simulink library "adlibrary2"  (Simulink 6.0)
settings: Solver=ode45  StartTime=0.0  StopTime=10.0  RelTol=1e-3
undefined symbols (not defined in the file or in its folder): adlibrary2, ADM, Bit, DDR, Generation, II, Location, Lower, SDRAM, SRAM, Width, XP, XPL, XRC, ZBT
libraries: xbsIndex_r3 x581, adlibrary2 x2
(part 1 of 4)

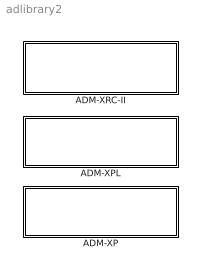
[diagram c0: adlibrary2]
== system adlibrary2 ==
  ADM-XP : Subsystem
  ADM-XPL : Subsystem
  ADM-XRC-II : Subsystem

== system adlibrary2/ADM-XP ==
  DDR SDRAM 1 : Subsystem  mask{memsize=1}
      mask prompts: memsize "Simulation RAM Size (Mb)"
      mask init:
      | as=get_param(gcb,'MaskIconUnits');
      | if (as(1)=='p')
      | 	im=imread('adbutton.jpg');s=get_param(gcb,'MaskDisplay');
      |     add_ad_icon(67,60);
      | else	
      | 	rm_ad_icon
      | end
  DDR SDRAM 2 : Subsystem  AncestorBlock=adlibrary2/ADM-XP/DDR SDRAM 1  mask{memsize=1}
      mask prompts: memsize "Simulation RAM Size (Mb)"
      mask init:
      | as=get_param(gcb,'MaskIconUnits');
      | if (as(1)=='p')
      | 	im=imread('adbutton.jpg');s=get_param(gcb,'MaskDisplay');
      |     add_ad_icon(67,60);
      | else	
      | 	rm_ad_icon
      | end
  DDRII SRAM 0 : Subsystem
  DDRII SRAM 1 : Subsystem
  DDRII SRAM 2 : Subsystem
  DDRII SRAM 3 : Subsystem
  XPL 32 Bit Interface : Subsystem  mask{program='load myprogram.txt', clock_ratio=1.5}
      mask prompts: program "Local Bus Script Program"; clock_ratio "Clock Ratio"
      mask init:
      | as=get_param(gcb,'MaskIconUnits');
      | if (as(1)=='p')
      | 	im=imread('adbutton.jpg');s=get_param(gcb,'MaskDisplay');
      |     add_ad_icon(74,56);
      | else	
      | 	rm_ad_icon
      | end
  XPL 64 Bit Interface : Subsystem  mask{program='load myprogram.txt', clock_ratio=1.5}
      mask prompts: program "Local Bus Script Program"; clock_ratio "Clock Ratio"
      mask init:
      | as=get_param(gcb,'MaskIconUnits');
      | if (as(1)=='p')
      | 	im=imread('adbutton.jpg');s=get_param(gcb,'MaskDisplay');
      |     add_ad_icon(74,56);
      | else	
      | 	rm_ad_icon
      | end

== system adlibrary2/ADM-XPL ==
  "DDR SDRAM " : Subsystem  mask{memsize=1}
      mask prompts: memsize "Simulation RAM Size (Mb)"
      mask init:
      | as=get_param(gcb,'MaskIconUnits');
      | if (as(1)=='p')
      | 	im=imread('adbutton.jpg');s=get_param(gcb,'MaskDisplay');
      |     add_ad_icon(67,60);
      | else	
      | 	rm_ad_icon
      | end
  XPL 32 Bit Interface : Subsystem  mask{program='load myprogram.txt', clock_ratio=1.5}
      mask prompts: program "Local Bus Script Program"; clock_ratio "Clock Ratio"
      mask init:
      | as=get_param(gcb,'MaskIconUnits');
      | if (as(1)=='p')
      | 	im=imread('adbutton.jpg');s=get_param(gcb,'MaskDisplay');
      |     add_ad_icon(74,56);
      | else	
      | 	rm_ad_icon
      | end
  XPL 64 Bit Interface : Subsystem  mask{program='load myprogram.txt', clock_ratio=1.5}
      mask prompts: program "Local Bus Script Program"; clock_ratio "Clock Ratio"
      mask init:
      | as=get_param(gcb,'MaskIconUnits');
      | if (as(1)=='p')
      | 	im=imread('adbutton.jpg');s=get_param(gcb,'MaskDisplay');
      |     add_ad_icon(74,56);
      | else	
      | 	rm_ad_icon
      | end
  ZBT SRAM 64 : Subsystem

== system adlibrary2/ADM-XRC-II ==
  PLX 32 Bit Interface : Subsystem  mask{program='load myprogram.txt', clock_ratio=1.5}
      mask prompts: program "Local Bus Script Program"; clock_ratio "Clock Ratio"
      mask init:
      | as=get_param(gcb,'MaskIconUnits');
      | if (as(1)=='p')
      | 	im=imread('adbutton.jpg');s=get_param(gcb,'MaskDisplay');
      |     add_ad_icon(74,56);
      | else	
      | 	rm_ad_icon
      | end
  "XRM DDR SDRAM " : Subsystem  mask{memsize=1}
      mask prompts: memsize "Simulation RAM Size (Mb)"
      mask init:
      | as=get_param(gcb,'MaskIconUnits');
      | if (as(1)=='p')
      | 	im=imread('adbutton.jpg');s=get_param(gcb,'MaskDisplay');
      |     add_ad_icon(67,60);
      | else	
      | 	rm_ad_icon
      | end
  ZBT SRAM 0 : Subsystem
  ZBT SRAM 1 : Subsystem  AncestorBlock=adlibrary2/ADM-XRC-II/ZBT SRAM 0
  ZBT SRAM 2 : Subsystem  AncestorBlock=adlibrary2/ADM-XRC-II/ZBT SRAM 0
  ZBT SRAM 3 : Subsystem  AncestorBlock=adlibrary2/ADM-XRC-II/ZBT SRAM 0
  ZBT SRAM 4 : Subsystem  AncestorBlock=adlibrary2/ADM-XRC-II/ZBT SRAM 0
  ZBT SRAM 5 : Subsystem  AncestorBlock=adlibrary2/ADM-XRC-II/ZBT SRAM 0

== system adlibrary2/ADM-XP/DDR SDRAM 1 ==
  cache_data_in : Inport  Port=1  LatchInput=off
  cache_addr : Inport  Port=2  LatchInput=off
  cache_write : Inport  Port=3  LatchInput=off
  ddr_page : Inport  Port=4  LatchInput=off
  ddr_addr : Inport  Port=5  LatchInput=off
  ddr_read : Inport  Port=6  LatchInput=off
  ddr_write : Inport  Port=7  LatchInput=off
  DDR SDRAM 32Bit Generation : Subsystem  AncestorBlock=adlibrary2/ADM-XPL/DDR SDRAM /DDR SDRAM 32Bit Generation
  DDR SDRAM 32bit Simulation : Subsystem  mask{memsize=memsize}
      mask prompts: memsize "Simulation Ram Size (Mb)"
  Simulation Multiplexer : xbsIndex_r3/Simulation Multiplexer  sim_sel=1  hw_sel=2
  Simulation Multiplexer1 : xbsIndex_r3/Simulation Multiplexer  sim_sel=1  hw_sel=2
  Simulation Multiplexer2 : xbsIndex_r3/Simulation Multiplexer  sim_sel=1  hw_sel=2
  cache_data_out : Outport
  ddr_busy : Outport  Port=2
  ddr_status : Outport  Port=3
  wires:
  cache_data_in/1 -> DDR SDRAM 32bit Simulation/1(cache_data_in), DDR SDRAM 32Bit Generation/1(cache_data_in)
  cache_addr/1 -> DDR SDRAM 32bit Simulation/2(cache_addr), DDR SDRAM 32Bit Generation/2(cache_addr)
  cache_write/1 -> DDR SDRAM 32bit Simulation/3(cache_write), DDR SDRAM 32Bit Generation/3(cache_write)
  ddr_page/1 -> DDR SDRAM 32bit Simulation/4(ddr_page), DDR SDRAM 32Bit Generation/4(ddr_page)
  ddr_addr/1 -> DDR SDRAM 32bit Simulation/5(ddr_addr), DDR SDRAM 32Bit Generation/5(ddr_addr)
  ddr_read/1 -> DDR SDRAM 32bit Simulation/6(ddr_read), DDR SDRAM 32Bit Generation/6(ddr_read)
  ddr_write/1 -> DDR SDRAM 32bit Simulation/7(ddr_write), DDR SDRAM 32Bit Generation/7(ddr_write)
  Simulation Multiplexer/1 -> cache_data_out/1
  Simulation Multiplexer1/1 -> ddr_busy/1
  Simulation Multiplexer2/1 -> ddr_status/1
  DDR SDRAM 32bit Simulation/3(ddr_status) -> Simulation Multiplexer2/1
  DDR SDRAM 32bit Simulation/2(ddr_busy) -> Simulation Multiplexer1/1
  DDR SDRAM 32bit Simulation/1(cache_data_out) -> Simulation Multiplexer/1
  DDR SDRAM 32Bit Generation/1(cache_data_out) -> Simulation Multiplexer/2
  DDR SDRAM 32Bit Generation/2(ddr_busy) -> Simulation Multiplexer1/2
  DDR SDRAM 32Bit Generation/3(ddr_status) -> Simulation Multiplexer2/2

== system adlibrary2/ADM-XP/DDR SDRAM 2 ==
  cache_data_in : Inport  Port=1  LatchInput=off
  cache_addr : Inport  Port=2  LatchInput=off
  cache_write : Inport  Port=3  LatchInput=off
  ddr_page : Inport  Port=4  LatchInput=off
  ddr_addr : Inport  Port=5  LatchInput=off
  ddr_read : Inport  Port=6  LatchInput=off
  ddr_write : Inport  Port=7  LatchInput=off
  DDR SDRAM 32Bit Generation : Subsystem  AncestorBlock=adlibrary2/ADM-XPL/DDR SDRAM /DDR SDRAM 32Bit Generation
  DDR SDRAM 32bit Simulation : Subsystem  mask{memsize=memsize}
      mask prompts: memsize "Simulation Ram Size (Mb)"
  Simulation Multiplexer : xbsIndex_r3/Simulation Multiplexer  sim_sel=1  hw_sel=2
  Simulation Multiplexer1 : xbsIndex_r3/Simulation Multiplexer  sim_sel=1  hw_sel=2
  Simulation Multiplexer2 : xbsIndex_r3/Simulation Multiplexer  sim_sel=1  hw_sel=2
  cache_data_out : Outport
  ddr_busy : Outport  Port=2
  ddr_status : Outport  Port=3
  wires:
  cache_data_in/1 -> DDR SDRAM 32bit Simulation/1(cache_data_in), DDR SDRAM 32Bit Generation/1(cache_data_in)
  cache_addr/1 -> DDR SDRAM 32bit Simulation/2(cache_addr), DDR SDRAM 32Bit Generation/2(cache_addr)
  cache_write/1 -> DDR SDRAM 32bit Simulation/3(cache_write), DDR SDRAM 32Bit Generation/3(cache_write)
  ddr_page/1 -> DDR SDRAM 32bit Simulation/4(ddr_page), DDR SDRAM 32Bit Generation/4(ddr_page)
  ddr_addr/1 -> DDR SDRAM 32bit Simulation/5(ddr_addr), DDR SDRAM 32Bit Generation/5(ddr_addr)
  ddr_read/1 -> DDR SDRAM 32bit Simulation/6(ddr_read), DDR SDRAM 32Bit Generation/6(ddr_read)
  ddr_write/1 -> DDR SDRAM 32bit Simulation/7(ddr_write), DDR SDRAM 32Bit Generation/7(ddr_write)
  Simulation Multiplexer/1 -> cache_data_out/1
  Simulation Multiplexer1/1 -> ddr_busy/1
  Simulation Multiplexer2/1 -> ddr_status/1
  DDR SDRAM 32bit Simulation/3(ddr_status) -> Simulation Multiplexer2/1
  DDR SDRAM 32bit Simulation/2(ddr_busy) -> Simulation Multiplexer1/1
  DDR SDRAM 32bit Simulation/1(cache_data_out) -> Simulation Multiplexer/1
  DDR SDRAM 32Bit Generation/1(cache_data_out) -> Simulation Multiplexer/2
  DDR SDRAM 32Bit Generation/2(ddr_busy) -> Simulation Multiplexer1/2
  DDR SDRAM 32Bit Generation/3(ddr_status) -> Simulation Multiplexer2/2

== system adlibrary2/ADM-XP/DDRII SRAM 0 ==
  d : Inport  Port=1  LatchInput=off
  a : Inport  Port=2  LatchInput=off
  w : Inport  Port=3  LatchInput=off
  r : Inport  Port=4  LatchInput=off
  be : Inport  Port=5  LatchInput=off
  DDRII SRAM Generation : Subsystem
  DDRII SRAM Simulation : Subsystem
  Delay : xbsIndex_r3/Delay  latency=2  reg_retiming=off  explicit_period=off  period=1  en=off  accept_only_valid=off  init_zero=on  dbl_ovrd=off  show_param=off
  Simulation Multiplexer : xbsIndex_r3/Simulation Multiplexer  sim_sel=1  hw_sel=2
  Simulation Multiplexer1 : xbsIndex_r3/Simulation Multiplexer  sim_sel=1  hw_sel=2
  q : Outport
  qv : Outport  Port=2
  read_pending : Outport  Port=3
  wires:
  be/1 -> DDRII SRAM Generation/5(be), DDRII SRAM Simulation/5(be)
  r/1 -> DDRII SRAM Simulation/4(r), DDRII SRAM Generation/4(r), Delay/1
  w/1 -> DDRII SRAM Generation/3(w), DDRII SRAM Simulation/3(w)
  a/1 -> DDRII SRAM Generation/2(a), DDRII SRAM Simulation/2(a)
  d/1 -> DDRII SRAM Generation/1(d), DDRII SRAM Simulation/1(d)
  DDRII SRAM Simulation/1(q) -> Simulation Multiplexer/1
  DDRII SRAM Generation/1(q) -> Simulation Multiplexer/2
  Simulation Multiplexer/1 -> q/1
  Delay/1 -> qv/1
  Simulation Multiplexer1/1 -> read_pending/1
  DDRII SRAM Generation/2(read_pending) -> Simulation Multiplexer1/2
  DDRII SRAM Simulation/2(qv) -> Simulation Multiplexer1/1

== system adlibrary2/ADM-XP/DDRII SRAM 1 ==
  d : Inport  Port=1  LatchInput=off
  a : Inport  Port=2  LatchInput=off
  w : Inport  Port=3  LatchInput=off
  r : Inport  Port=4  LatchInput=off
  be : Inport  Port=5  LatchInput=off
  DDRII SRAM Generation : Subsystem
  DDRII SRAM Simulation : Subsystem
  Delay : xbsIndex_r3/Delay  latency=2  reg_retiming=off  explicit_period=off  period=1  en=off  accept_only_valid=off  init_zero=on  dbl_ovrd=off  show_param=off
  Simulation Multiplexer : xbsIndex_r3/Simulation Multiplexer  sim_sel=1  hw_sel=2
  Simulation Multiplexer1 : xbsIndex_r3/Simulation Multiplexer  sim_sel=1  hw_sel=2
  q : Outport
  qv : Outport  Port=2
  read_pending : Outport  Port=3
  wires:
  DDRII SRAM Simulation/2(qv) -> Simulation Multiplexer1/1
  DDRII SRAM Generation/2(read_pending) -> Simulation Multiplexer1/2
  Simulation Multiplexer1/1 -> read_pending/1
  Delay/1 -> qv/1
  Simulation Multiplexer/1 -> q/1
  DDRII SRAM Generation/1(q) -> Simulation Multiplexer/2
  DDRII SRAM Simulation/1(q) -> Simulation Multiplexer/1
  d/1 -> DDRII SRAM Simulation/1(d), DDRII SRAM Generation/1(d)
  a/1 -> DDRII SRAM Simulation/2(a), DDRII SRAM Generation/2(a)
  w/1 -> DDRII SRAM Simulation/3(w), DDRII SRAM Generation/3(w)
  r/1 -> Delay/1, DDRII SRAM Generation/4(r), DDRII SRAM Simulation/4(r)
  be/1 -> DDRII SRAM Simulation/5(be), DDRII SRAM Generation/5(be)

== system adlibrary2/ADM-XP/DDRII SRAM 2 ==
  d : Inport  Port=1  LatchInput=off
  a : Inport  Port=2  LatchInput=off
  w : Inport  Port=3  LatchInput=off
  r : Inport  Port=4  LatchInput=off
  be : Inport  Port=5  LatchInput=off
  DDRII SRAM Generation : Subsystem
  DDRII SRAM Simulation : Subsystem
  Delay : xbsIndex_r3/Delay  latency=2  reg_retiming=off  explicit_period=off  period=1  en=off  accept_only_valid=off  init_zero=on  dbl_ovrd=off  show_param=off
  Simulation Multiplexer : xbsIndex_r3/Simulation Multiplexer  sim_sel=1  hw_sel=2
  Simulation Multiplexer1 : xbsIndex_r3/Simulation Multiplexer  sim_sel=1  hw_sel=2
  q : Outport
  qv : Outport  Port=2
  read_pending : Outport  Port=3
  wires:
  be/1 -> DDRII SRAM Generation/5(be), DDRII SRAM Simulation/5(be)
  r/1 -> DDRII SRAM Simulation/4(r), DDRII SRAM Generation/4(r), Delay/1
  w/1 -> DDRII SRAM Generation/3(w), DDRII SRAM Simulation/3(w)
  a/1 -> DDRII SRAM Generation/2(a), DDRII SRAM Simulation/2(a)
  d/1 -> DDRII SRAM Generation/1(d), DDRII SRAM Simulation/1(d)
  DDRII SRAM Simulation/1(q) -> Simulation Multiplexer/1
  DDRII SRAM Generation/1(q) -> Simulation Multiplexer/2
  Simulation Multiplexer/1 -> q/1
  Delay/1 -> qv/1
  Simulation Multiplexer1/1 -> read_pending/1
  DDRII SRAM Generation/2(read_pending) -> Simulation Multiplexer1/2
  DDRII SRAM Simulation/2(qv) -> Simulation Multiplexer1/1

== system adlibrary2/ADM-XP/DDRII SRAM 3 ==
  d : Inport  Port=1  LatchInput=off
  a : Inport  Port=2  LatchInput=off
  w : Inport  Port=3  LatchInput=off
  r : Inport  Port=4  LatchInput=off
  be : Inport  Port=5  LatchInput=off
  DDRII SRAM Generation : Subsystem
  DDRII SRAM Simulation : Subsystem
  Delay : xbsIndex_r3/Delay  latency=2  reg_retiming=off  explicit_period=off  period=1  en=off  accept_only_valid=off  init_zero=on  dbl_ovrd=off  show_param=off
  Simulation Multiplexer : xbsIndex_r3/Simulation Multiplexer  sim_sel=1  hw_sel=2
  Simulation Multiplexer1 : xbsIndex_r3/Simulation Multiplexer  sim_sel=1  hw_sel=2
  q : Outport
  qv : Outport  Port=2
  read_pending : Outport  Port=3
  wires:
  be/1 -> DDRII SRAM Generation/5(be), DDRII SRAM Simulation/5(be)
  r/1 -> DDRII SRAM Simulation/4(r), DDRII SRAM Generation/4(r), Delay/1
  w/1 -> DDRII SRAM Generation/3(w), DDRII SRAM Simulation/3(w)
  a/1 -> DDRII SRAM Generation/2(a), DDRII SRAM Simulation/2(a)
  d/1 -> DDRII SRAM Generation/1(d), DDRII SRAM Simulation/1(d)
  DDRII SRAM Simulation/1(q) -> Simulation Multiplexer/1
  DDRII SRAM Generation/1(q) -> Simulation Multiplexer/2
  Simulation Multiplexer/1 -> q/1
  Delay/1 -> qv/1
  Simulation Multiplexer1/1 -> read_pending/1
  DDRII SRAM Generation/2(read_pending) -> Simulation Multiplexer1/2
  DDRII SRAM Simulation/2(qv) -> Simulation Multiplexer1/1

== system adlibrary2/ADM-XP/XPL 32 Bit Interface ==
  Data_Read : Inport  Port=1  LatchInput=off
  Ack : Inport  Port=2  LatchInput=off
  Status : Inport  Port=3  LatchInput=off
  Read IFIFO : Inport  Port=4  LatchInput=off
  Write OFIFO : Inport  Port=5  LatchInput=off
  OFIFO_Data : Inport  Port=6  LatchInput=off
  Simulation Multiplexer{,1..8} (9 alike) : xbsIndex_r3/Simulation Multiplexer  sim_sel=1  hw_sel=2
  XPL 32Bit Generation : Subsystem
  XPL 32Bit Simulation : Subsystem  mask{program=program, clock_ratio=clock_ratio}
      mask prompts: program "Local Bus Script Program"; clock_ratio "Clock Ratio"
  Data_Write : Outport
  Addr : Outport  Port=2
  BE : Outport  Port=3
  Write : Outport  Port=4
  Read : Outport  Port=5
  Control : Outport  Port=6
  IFIFO_Data : Outport  Port=7
  IFIFO_Empty : Outport  Port=8
  OFIFO_Full : Outport  Port=9
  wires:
  XPL 32Bit Generation/3(BE) -> Simulation Multiplexer1/2
  XPL 32Bit Simulation/3(BE) -> Simulation Multiplexer1/1
  XPL 32Bit Simulation/2(Addr) -> Simulation Multiplexer8/1
  Simulation Multiplexer8/1 -> Addr/1
  XPL 32Bit Simulation/4(Write) -> Simulation Multiplexer2/1
  XPL 32Bit Simulation/5(Read) -> Simulation Multiplexer3/1
  XPL 32Bit Simulation/6(Control) -> Simulation Multiplexer4/1
  XPL 32Bit Simulation/7(IFIFO_Data) -> Simulation Multiplexer5/1
  XPL 32Bit Simulation/8(IFIFO_Empty) -> Simulation Multiplexer6/1
  Simulation Multiplexer/1 -> Data_Write/1
  Simulation Multiplexer1/1 -> BE/1
  Simulation Multiplexer2/1 -> Write/1
  Simulation Multiplexer3/1 -> Read/1
  Simulation Multiplexer4/1 -> Control/1
  Simulation Multiplexer5/1 -> IFIFO_Data/1
  Simulation Multiplexer6/1 -> IFIFO_Empty/1
  Simulation Multiplexer7/1 -> OFIFO_Full/1
  XPL 32Bit Generation/9(OFIFO_Full) -> Simulation Multiplexer7/2
  XPL 32Bit Generation/8(IFIFO_Empty) -> Simulation Multiplexer6/2
  XPL 32Bit Generation/7(IFIFO_Data) -> Simulation Multiplexer5/2
  XPL 32Bit Generation/6(Control) -> Simulation Multiplexer4/2
  XPL 32Bit Generation/5(Read) -> Simulation Multiplexer3/2
  XPL 32Bit Generation/4(Write) -> Simulation Multiplexer2/2
  XPL 32Bit Generation/2(Addr) -> Simulation Multiplexer8/2
  XPL 32Bit Generation/1(Data_Write) -> Simulation Multiplexer/2
  XPL 32Bit Simulation/1(Data_Write) -> Simulation Multiplexer/1
  XPL 32Bit Simulation/9(OFIFO_Full) -> Simulation Multiplexer7/1
  Data_Read/1 -> XPL 32Bit Simulation/1(Data_Read), XPL 32Bit Generation/1(Data_Read)
  Ack/1 -> XPL 32Bit Simulation/2(Ack), XPL 32Bit Generation/2(Ack)
  Status/1 -> XPL 32Bit Simulation/3(Status), XPL 32Bit Generation/3(Status)
  Read IFIFO/1 -> XPL 32Bit Simulation/4(Read IFIFO), XPL 32Bit Generation/4(Read IFIFO)
  Write OFIFO/1 -> XPL 32Bit Simulation/5(Write OFIFO), XPL 32Bit Generation/5(Write OFIFO)
  OFIFO_Data/1 -> XPL 32Bit Simulation/6(OFIFO_Data), XPL 32Bit Generation/6(OFIFO_Data)

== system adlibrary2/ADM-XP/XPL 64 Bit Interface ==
  Data_Read : Inport  Port=1  LatchInput=off
  Ack : Inport  Port=2  LatchInput=off
  Status : Inport  Port=3  LatchInput=off
  Read IFIFO : Inport  Port=4  LatchInput=off
  Write OFIFO : Inport  Port=5  LatchInput=off
  OFIFO_Data : Inport  Port=6  LatchInput=off
  Simulation Multiplexer{,1..8} (9 alike) : xbsIndex_r3/Simulation Multiplexer  sim_sel=1  hw_sel=2
  XPL 64Bit Generation : Subsystem
  XPL 64Bit Simulation : Subsystem  mask{program=program, clock_ratio=clock_ratio}
      mask prompts: program "Local Bus Script Program"; clock_ratio "Clock Ratio"
  Data_Write : Outport
  Addr : Outport  Port=2
  BE : Outport  Port=3
  Write : Outport  Port=4
  Read : Outport  Port=5
  Control : Outport  Port=6
  IFIFO_Data : Outport  Port=7
  IFIFO_Empty : Outport  Port=8
  OFIFO_Full : Outport  Port=9
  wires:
  XPL 64Bit Simulation/3(BE) -> Simulation Multiplexer8/1
  XPL 64Bit Generation/3(BE) -> Simulation Multiplexer8/2
  Simulation Multiplexer8/1 -> BE/1
  OFIFO_Data/1 -> XPL 64Bit Generation/6(OFIFO_Data), XPL 64Bit Simulation/6(OFIFO_Data)
  Write OFIFO/1 -> XPL 64Bit Generation/5(Write OFIFO), XPL 64Bit Simulation/5(Write OFIFO)
  Read IFIFO/1 -> XPL 64Bit Generation/4(Read IFIFO), XPL 64Bit Simulation/4(Read IFIFO)
  Status/1 -> XPL 64Bit Generation/3(Status), XPL 64Bit Simulation/3(Status)
  Ack/1 -> XPL 64Bit Generation/2(Ack), XPL 64Bit Simulation/2(Ack)
  Data_Read/1 -> XPL 64Bit Generation/1(Data_Read), XPL 64Bit Simulation/1(Data_Read)
  XPL 64Bit Simulation/9(OFIFO_Full) -> Simulation Multiplexer7/1
  XPL 64Bit Simulation/8(IFIFO_Empty) -> Simulation Multiplexer6/1
  XPL 64Bit Simulation/7(IFIFO_Data) -> Simulation Multiplexer5/1
  XPL 64Bit Simulation/6(Control) -> Simulation Multiplexer4/1
  XPL 64Bit Simulation/5(Read) -> Simulation Multiplexer3/1
  XPL 64Bit Simulation/4(Write) -> Simulation Multiplexer2/1
  XPL 64Bit Simulation/2(Addr) -> Simulation Multiplexer1/1
  XPL 64Bit Simulation/1(Data_Write) -> Simulation Multiplexer/1
  XPL 64Bit Generation/1(Data_Write) -> Simulation Multiplexer/2
  XPL 64Bit Generation/2(Addr) -> Simulation Multiplexer1/2
  XPL 64Bit Generation/4(Write) -> Simulation Multiplexer2/2
  XPL 64Bit Generation/5(Read) -> Simulation Multiplexer3/2
  XPL 64Bit Generation/6(Control) -> Simulation Multiplexer4/2
  XPL 64Bit Generation/7(IFIFO_Data) -> Simulation Multiplexer5/2
  XPL 64Bit Generation/8(IFIFO_Empty) -> Simulation Multiplexer6/2
  XPL 64Bit Generation/9(OFIFO_Full) -> Simulation Multiplexer7/2
  Simulation Multiplexer7/1 -> OFIFO_Full/1
  Simulation Multiplexer6/1 -> IFIFO_Empty/1
  Simulation Multiplexer5/1 -> IFIFO_Data/1
  Simulation Multiplexer4/1 -> Control/1
  Simulation Multiplexer3/1 -> Read/1
  Simulation Multiplexer2/1 -> Write/1
  Simulation Multiplexer1/1 -> Addr/1
  Simulation Multiplexer/1 -> Data_Write/1

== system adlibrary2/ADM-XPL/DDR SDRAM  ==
  cache_data_in : Inport  Port=1  LatchInput=off
  cache_addr : Inport  Port=2  LatchInput=off
  cache_write : Inport  Port=3  LatchInput=off
  ddr_page : Inport  Port=4  LatchInput=off
  ddr_addr : Inport  Port=5  LatchInput=off
  ddr_read : Inport  Port=6  LatchInput=off
  ddr_write : Inport  Port=7  LatchInput=off
  DDR SDRAM 32Bit Generation : Subsystem
  DDR SDRAM 32bit Simulation : Subsystem  mask{memsize=memsize}
      mask prompts: memsize "Simulation Ram Size (Mb)"
  Simulation Multiplexer : xbsIndex_r3/Simulation Multiplexer  sim_sel=1  hw_sel=2
  Simulation Multiplexer1 : xbsIndex_r3/Simulation Multiplexer  sim_sel=1  hw_sel=2
  Simulation Multiplexer2 : xbsIndex_r3/Simulation Multiplexer  sim_sel=1  hw_sel=2
  cache_data_out : Outport
  ddr_busy : Outport  Port=2
  ddr_status : Outport  Port=3
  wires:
  DDR SDRAM 32Bit Generation/3(ddr_status) -> Simulation Multiplexer2/2
  DDR SDRAM 32Bit Generation/2(ddr_busy) -> Simulation Multiplexer1/2
  DDR SDRAM 32Bit Generation/1(cache_data_out) -> Simulation Multiplexer/2
  DDR SDRAM 32bit Simulation/1(cache_data_out) -> Simulation Multiplexer/1
  DDR SDRAM 32bit Simulation/2(ddr_busy) -> Simulation Multiplexer1/1
  DDR SDRAM 32bit Simulation/3(ddr_status) -> Simulation Multiplexer2/1
  Simulation Multiplexer2/1 -> ddr_status/1
  Simulation Multiplexer1/1 -> ddr_busy/1
  Simulation Multiplexer/1 -> cache_data_out/1
  ddr_write/1 -> DDR SDRAM 32bit Simulation/7(ddr_write), DDR SDRAM 32Bit Generation/7(ddr_write)
  ddr_read/1 -> DDR SDRAM 32bit Simulation/6(ddr_read), DDR SDRAM 32Bit Generation/6(ddr_read)
  ddr_addr/1 -> DDR SDRAM 32Bit Generation/5(ddr_addr), DDR SDRAM 32bit Simulation/5(ddr_addr)
  ddr_page/1 -> DDR SDRAM 32Bit Generation/4(ddr_page), DDR SDRAM 32bit Simulation/4(ddr_page)
  cache_write/1 -> DDR SDRAM 32Bit Generation/3(cache_write), DDR SDRAM 32bit Simulation/3(cache_write)
  cache_addr/1 -> DDR SDRAM 32Bit Generation/2(cache_addr), DDR SDRAM 32bit Simulation/2(cache_addr)
  cache_data_in/1 -> DDR SDRAM 32Bit Generation/1(cache_data_in), DDR SDRAM 32bit Simulation/1(cache_data_in)

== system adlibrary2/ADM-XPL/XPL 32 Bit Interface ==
  Data_Read : Inport  Port=1  LatchInput=off
  Ack : Inport  Port=2  LatchInput=off
  Status : Inport  Port=3  LatchInput=off
  Read IFIFO : Inport  Port=4  LatchInput=off
  Write OFIFO : Inport  Port=5  LatchInput=off
  OFIFO_Data : Inport  Port=6  LatchInput=off
  Simulation Multiplexer{,1..8} (9 alike) : xbsIndex_r3/Simulation Multiplexer  sim_sel=1  hw_sel=2
  XPL 32Bit Generation : Subsystem
  XPL 32Bit Simulation : Subsystem  mask{program=program, clock_ratio=clock_ratio}
      mask prompts: program "Local Bus Script Program"; clock_ratio "Clock Ratio"
  Data_Write : Outport
  Addr : Outport  Port=2
  BE : Outport  Port=3
  Write : Outport  Port=4
  Read : Outport  Port=5
  Control : Outport  Port=6
  IFIFO_Data : Outport  Port=7
  IFIFO_Empty : Outport  Port=8
  OFIFO_Full : Outport  Port=9
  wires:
  OFIFO_Data/1 -> XPL 32Bit Generation/6(OFIFO_Data), XPL 32Bit Simulation/6(OFIFO_Data)
  Write OFIFO/1 -> XPL 32Bit Generation/5(Write OFIFO), XPL 32Bit Simulation/5(Write OFIFO)
  Read IFIFO/1 -> XPL 32Bit Generation/4(Read IFIFO), XPL 32Bit Simulation/4(Read IFIFO)
  Status/1 -> XPL 32Bit Generation/3(Status), XPL 32Bit Simulation/3(Status)
  Ack/1 -> XPL 32Bit Generation/2(Ack), XPL 32Bit Simulation/2(Ack)
  Data_Read/1 -> XPL 32Bit Generation/1(Data_Read), XPL 32Bit Simulation/1(Data_Read)
  XPL 32Bit Simulation/9(OFIFO_Full) -> Simulation Multiplexer7/1
  XPL 32Bit Simulation/1(Data_Write) -> Simulation Multiplexer/1
  XPL 32Bit Generation/1(Data_Write) -> Simulation Multiplexer/2
  XPL 32Bit Generation/2(Addr) -> Simulation Multiplexer8/2
  XPL 32Bit Generation/4(Write) -> Simulation Multiplexer2/2
  XPL 32Bit Generation/5(Read) -> Simulation Multiplexer3/2
  XPL 32Bit Generation/6(Control) -> Simulation Multiplexer4/2
  XPL 32Bit Generation/7(IFIFO_Data) -> Simulation Multiplexer5/2
  XPL 32Bit Generation/8(IFIFO_Empty) -> Simulation Multiplexer6/2
  XPL 32Bit Generation/9(OFIFO_Full) -> Simulation Multiplexer7/2
  Simulation Multiplexer7/1 -> OFIFO_Full/1
  Simulation Multiplexer6/1 -> IFIFO_Empty/1
  Simulation Multiplexer5/1 -> IFIFO_Data/1
  Simulation Multiplexer4/1 -> Control/1
  Simulation Multiplexer3/1 -> Read/1
  Simulation Multiplexer2/1 -> Write/1
  Simulation Multiplexer1/1 -> BE/1
  Simulation Multiplexer/1 -> Data_Write/1
  XPL 32Bit Simulation/8(IFIFO_Empty) -> Simulation Multiplexer6/1
  XPL 32Bit Simulation/7(IFIFO_Data) -> Simulation Multiplexer5/1
  XPL 32Bit Simulation/6(Control) -> Simulation Multiplexer4/1
  XPL 32Bit Simulation/5(Read) -> Simulation Multiplexer3/1
  XPL 32Bit Simulation/4(Write) -> Simulation Multiplexer2/1
  Simulation Multiplexer8/1 -> Addr/1
  XPL 32Bit Simulation/2(Addr) -> Simulation Multiplexer8/1
  XPL 32Bit Simulation/3(BE) -> Simulation Multiplexer1/1
  XPL 32Bit Generation/3(BE) -> Simulation Multiplexer1/2

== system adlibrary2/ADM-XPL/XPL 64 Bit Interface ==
  Data_Read : Inport  Port=1  LatchInput=off
  Ack : Inport  Port=2  LatchInput=off
  Status : Inport  Port=3  LatchInput=off
  Read IFIFO : Inport  Port=4  LatchInput=off
  Write OFIFO : Inport  Port=5  LatchInput=off
  OFIFO_Data : Inport  Port=6  LatchInput=off
  Simulation Multiplexer{,1..8} (9 alike) : xbsIndex_r3/Simulation Multiplexer  sim_sel=1  hw_sel=2
  XPL 64Bit Generation : Subsystem
  XPL 64Bit Simulation : Subsystem  mask{program=program, clock_ratio=clock_ratio}
      mask prompts: program "Local Bus Script Program"; clock_ratio "Clock Ratio"
  Data_Write : Outport
  Addr : Outport  Port=2
  BE : Outport  Port=3
  Write : Outport  Port=4
  Read : Outport  Port=5
  Control : Outport  Port=6
  IFIFO_Data : Outport  Port=7
  IFIFO_Empty : Outport  Port=8
  OFIFO_Full : Outport  Port=9
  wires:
  Simulation Multiplexer/1 -> Data_Write/1
  Simulation Multiplexer1/1 -> Addr/1
  Simulation Multiplexer2/1 -> Write/1
  Simulation Multiplexer3/1 -> Read/1
  Simulation Multiplexer4/1 -> Control/1
  Simulation Multiplexer5/1 -> IFIFO_Data/1
  Simulation Multiplexer6/1 -> IFIFO_Empty/1
  Simulation Multiplexer7/1 -> OFIFO_Full/1
  XPL 64Bit Generation/9(OFIFO_Full) -> Simulation Multiplexer7/2
  XPL 64Bit Generation/8(IFIFO_Empty) -> Simulation Multiplexer6/2
  XPL 64Bit Generation/7(IFIFO_Data) -> Simulation Multiplexer5/2
  XPL 64Bit Generation/6(Control) -> Simulation Multiplexer4/2
  XPL 64Bit Generation/5(Read) -> Simulation Multiplexer3/2
  XPL 64Bit Generation/4(Write) -> Simulation Multiplexer2/2
  XPL 64Bit Generation/2(Addr) -> Simulation Multiplexer1/2
  XPL 64Bit Generation/1(Data_Write) -> Simulation Multiplexer/2
  XPL 64Bit Simulation/1(Data_Write) -> Simulation Multiplexer/1
  XPL 64Bit Simulation/2(Addr) -> Simulation Multiplexer1/1
  XPL 64Bit Simulation/4(Write) -> Simulation Multiplexer2/1
  XPL 64Bit Simulation/5(Read) -> Simulation Multiplexer3/1
  XPL 64Bit Simulation/6(Control) -> Simulation Multiplexer4/1
  XPL 64Bit Simulation/7(IFIFO_Data) -> Simulation Multiplexer5/1
  XPL 64Bit Simulation/8(IFIFO_Empty) -> Simulation Multiplexer6/1
  XPL 64Bit Simulation/9(OFIFO_Full) -> Simulation Multiplexer7/1
  Data_Read/1 -> XPL 64Bit Simulation/1(Data_Read), XPL 64Bit Generation/1(Data_Read)
  Ack/1 -> XPL 64Bit Simulation/2(Ack), XPL 64Bit Generation/2(Ack)
  Status/1 -> XPL 64Bit Simulation/3(Status), XPL 64Bit Generation/3(Status)
  Read IFIFO/1 -> XPL 64Bit Simulation/4(Read IFIFO), XPL 64Bit Generation/4(Read IFIFO)
  Write OFIFO/1 -> XPL 64Bit Simulation/5(Write OFIFO), XPL 64Bit Generation/5(Write OFIFO)
  OFIFO_Data/1 -> XPL 64Bit Simulation/6(OFIFO_Data), XPL 64Bit Generation/6(OFIFO_Data)
  Simulation Multiplexer8/1 -> BE/1
  XPL 64Bit Generation/3(BE) -> Simulation Multiplexer8/2
  XPL 64Bit Simulation/3(BE) -> Simulation Multiplexer8/1

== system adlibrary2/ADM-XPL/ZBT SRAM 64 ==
  d : Inport  Port=1  LatchInput=off
  a : Inport  Port=2  LatchInput=off
  w : Inport  Port=3  LatchInput=off
  r : Inport  Port=4  LatchInput=off
  be : Inport  Port=5  LatchInput=off
  Simulation Multiplexer : xbsIndex_r3/Simulation Multiplexer  sim_sel=1  hw_sel=2
  Simulation Multiplexer1 : xbsIndex_r3/Simulation Multiplexer  sim_sel=1  hw_sel=2
  ZBT SRAM 64Bit Generation : Subsystem
  ZBT SRAM 64bit Simulation : Subsystem
  q : Outport
  qv : Outport  Port=2
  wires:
  Simulation Multiplexer/1 -> q/1
  ZBT SRAM 64Bit Generation/1(q) -> Simulation Multiplexer/2
  ZBT SRAM 64bit Simulation/1(q) -> Simulation Multiplexer/1
  d/1 -> ZBT SRAM 64bit Simulation/1(d), ZBT SRAM 64Bit Generation/1(d)
  a/1 -> ZBT SRAM 64bit Simulation/2(a), ZBT SRAM 64Bit Generation/2(a)
  w/1 -> ZBT SRAM 64bit Simulation/3(w), ZBT SRAM 64Bit Generation/3(w)
  Simulation Multiplexer1/1 -> qv/1
  r/1 -> ZBT SRAM 64bit Simulation/4(r), ZBT SRAM 64Bit Generation/4(r)
  ZBT SRAM 64bit Simulation/2(qv) -> Simulation Multiplexer1/1
  ZBT SRAM 64Bit Generation/2(qv) -> Simulation Multiplexer1/2
  be/1 -> ZBT SRAM 64bit Simulation/5(be), ZBT SRAM 64Bit Generation/5(be)

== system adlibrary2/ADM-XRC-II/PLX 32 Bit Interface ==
  Data_Read : Inport  Port=1  LatchInput=off
  Ack : Inport  Port=2  LatchInput=off
  Status : Inport  Port=3  LatchInput=off
  Read IFIFO : Inport  Port=4  LatchInput=off
  Write OFIFO : Inport  Port=5  LatchInput=off
  OFIFO_Data : Inport  Port=6  LatchInput=off
  PLX 32Bit Generation : Subsystem
  PLX 32Bit Simulation : Subsystem  mask{program=program, clock_ratio=clock_ratio}
      mask prompts: program "Local Bus Script Program"; clock_ratio "Clock Ratio"
  Simulation Multiplexer{,1..8} (9 alike) : xbsIndex_r3/Simulation Multiplexer  sim_sel=1  hw_sel=2
  Data_Write : Outport
  Addr : Outport  Port=2
  BE : Outport  Port=3
  Write : Outport  Port=4
  Read : Outport  Port=5
  Control : Outport  Port=6
  IFIFO_Data : Outport  Port=7
  IFIFO_Empty : Outport  Port=8
  OFIFO_Full : Outport  Port=9
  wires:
  Data_Read/1 -> PLX 32Bit Generation/1(Data_Read), PLX 32Bit Simulation/1(Data_Read)
  Ack/1 -> PLX 32Bit Generation/2(Ack), PLX 32Bit Simulation/2(Ack)
  Status/1 -> PLX 32Bit Generation/3(Status), PLX 32Bit Simulation/3(Status)
  Read IFIFO/1 -> PLX 32Bit Generation/4(Read IFIFO), PLX 32Bit Simulation/4(Read IFIFO)
  Write OFIFO/1 -> PLX 32Bit Generation/5(Write OFIFO), PLX 32Bit Simulation/5(Write OFIFO)
  OFIFO_Data/1 -> PLX 32Bit Generation/6(OFIFO_Data), PLX 32Bit Simulation/6(OFIFO_Data)
  Simulation Multiplexer/1 -> Data_Write/1
  Simulation Multiplexer1/1 -> Addr/1
  Simulation Multiplexer2/1 -> Write/1
  Simulation Multiplexer3/1 -> Read/1
  Simulation Multiplexer4/1 -> Control/1
  Simulation Multiplexer5/1 -> IFIFO_Data/1
  Simulation Multiplexer6/1 -> IFIFO_Empty/1
  Simulation Multiplexer7/1 -> OFIFO_Full/1
  PLX 32Bit Generation/9(OFIFO_Full) -> Simulation Multiplexer7/2
  PLX 32Bit Generation/8(IFIFO_Empty) -> Simulation Multiplexer6/2
  PLX 32Bit Generation/7(IFIFO_Data) -> Simulation Multiplexer5/2
  PLX 32Bit Generation/6(Control) -> Simulation Multiplexer4/2
  PLX 32Bit Generation/5(Read) -> Simulation Multiplexer3/2
  PLX 32Bit Generation/4(Write) -> Simulation Multiplexer2/2
  PLX 32Bit Generation/2(Addr) -> Simulation Multiplexer1/2
  PLX 32Bit Generation/1(Data_Write) -> Simulation Multiplexer/2
  PLX 32Bit Simulation/1(Data_Write) -> Simulation Multiplexer/1
  PLX 32Bit Simulation/2(Addr) -> Simulation Multiplexer1/1
  PLX 32Bit Simulation/4(Write) -> Simulation Multiplexer2/1
  PLX 32Bit Simulation/5(Read) -> Simulation Multiplexer3/1
  PLX 32Bit Simulation/6(Control) -> Simulation Multiplexer4/1
  PLX 32Bit Simulation/7(IFIFO_Data) -> Simulation Multiplexer5/1
  PLX 32Bit Simulation/8(IFIFO_Empty) -> Simulation Multiplexer6/1
  PLX 32Bit Simulation/9(OFIFO_Full) -> Simulation Multiplexer7/1
  Simulation Multiplexer8/1 -> BE/1
  PLX 32Bit Generation/3(BE) -> Simulation Multiplexer8/2
  PLX 32Bit Simulation/3(BE) -> Simulation Multiplexer8/1

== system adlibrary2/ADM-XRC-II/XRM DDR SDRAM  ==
  cache_data_in : Inport  Port=1  LatchInput=off
  cache_addr : Inport  Port=2  LatchInput=off
  cache_write : Inport  Port=3  LatchInput=off
  ddr_page : Inport  Port=4  LatchInput=off
  ddr_addr : Inport  Port=5  LatchInput=off
  ddr_read : Inport  Port=6  LatchInput=off
  ddr_write : Inport  Port=7  LatchInput=off
  DDR SDRAM 64Bit Generation : Subsystem
  DDR SDRAM 64bit Simulation : Subsystem  mask{memsize=memsize}
      mask prompts: memsize "Simulation Ram Size (Mb)"
  Simulation Multiplexer : xbsIndex_r3/Simulation Multiplexer  sim_sel=1  hw_sel=2
  Simulation Multiplexer1 : xbsIndex_r3/Simulation Multiplexer  sim_sel=1  hw_sel=2
  Simulation Multiplexer2 : xbsIndex_r3/Simulation Multiplexer  sim_sel=1  hw_sel=2
  cache_data_out : Outport
  ddr_busy : Outport  Port=2
  ddr_status : Outport  Port=3
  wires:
  cache_data_in/1 -> DDR SDRAM 64bit Simulation/1(cache_data_in), DDR SDRAM 64Bit Generation/1(cache_data_in)
  cache_addr/1 -> DDR SDRAM 64bit Simulation/2(cache_addr), DDR SDRAM 64Bit Generation/2(cache_addr)
  cache_write/1 -> DDR SDRAM 64bit Simulation/3(cache_write), DDR SDRAM 64Bit Generation/3(cache_write)
  ddr_page/1 -> DDR SDRAM 64bit Simulation/4(ddr_page), DDR SDRAM 64Bit Generation/4(ddr_page)
  ddr_addr/1 -> DDR SDRAM 64bit Simulation/5(ddr_addr), DDR SDRAM 64Bit Generation/5(ddr_addr)
  ddr_read/1 -> DDR SDRAM 64Bit Generation/6(ddr_read), DDR SDRAM 64bit Simulation/6(ddr_read)
  ddr_write/1 -> DDR SDRAM 64Bit Generation/7(ddr_write), DDR SDRAM 64bit Simulation/7(ddr_write)
  Simulation Multiplexer/1 -> cache_data_out/1
  Simulation Multiplexer1/1 -> ddr_busy/1
  Simulation Multiplexer2/1 -> ddr_status/1
  DDR SDRAM 64bit Simulation/3(ddr_status) -> Simulation Multiplexer2/1
  DDR SDRAM 64bit Simulation/2(ddr_busy) -> Simulation Multiplexer1/1
  DDR SDRAM 64bit Simulation/1(cache_data_out) -> Simulation Multiplexer/1
  DDR SDRAM 64Bit Generation/1(cache_data_out) -> Simulation Multiplexer/2
  DDR SDRAM 64Bit Generation/2(ddr_busy) -> Simulation Multiplexer1/2
  DDR SDRAM 64Bit Generation/3(ddr_status) -> Simulation Multiplexer2/2

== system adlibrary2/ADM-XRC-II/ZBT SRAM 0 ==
  d : Inport  Port=1  LatchInput=off
  a : Inport  Port=2  LatchInput=off
  w : Inport  Port=3  LatchInput=off
  r : Inport  Port=4  LatchInput=off
  be : Inport  Port=5  LatchInput=off
  Simulation Multiplexer : xbsIndex_r3/Simulation Multiplexer  sim_sel=1  hw_sel=2
  Simulation Multiplexer1 : xbsIndex_r3/Simulation Multiplexer  sim_sel=1  hw_sel=2
  ZBT SRAM 32Bit Generation : Subsystem
  ZBT SRAM 32Bit Simulation : Subsystem
  q : Outport
  qv : Outport  Port=2
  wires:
  r/1 -> ZBT SRAM 32Bit Generation/4(r), ZBT SRAM 32Bit Simulation/4(r)
  w/1 -> ZBT SRAM 32Bit Generation/3(w), ZBT SRAM 32Bit Simulation/3(w)
  a/1 -> ZBT SRAM 32Bit Generation/2(a), ZBT SRAM 32Bit Simulation/2(a)
  d/1 -> ZBT SRAM 32Bit Generation/1(d), ZBT SRAM 32Bit Simulation/1(d)
  ZBT SRAM 32Bit Simulation/2(qv) -> Simulation Multiplexer1/1
  ZBT SRAM 32Bit Simulation/1(q) -> Simulation Multiplexer/1
  ZBT SRAM 32Bit Generation/1(q) -> Simulation Multiplexer/2
  ZBT SRAM 32Bit Generation/2(qv) -> Simulation Multiplexer1/2
  Simulation Multiplexer1/1 -> qv/1
  Simulation Multiplexer/1 -> q/1
  be/1 -> ZBT SRAM 32Bit Simulation/5(be), ZBT SRAM 32Bit Generation/5(be)

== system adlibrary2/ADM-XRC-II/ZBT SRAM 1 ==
  d : Inport  Port=1  LatchInput=off
  a : Inport  Port=2  LatchInput=off
  w : Inport  Port=3  LatchInput=off
  r : Inport  Port=4  LatchInput=off
  be : Inport  Port=5  LatchInput=off
  Simulation Multiplexer : xbsIndex_r3/Simulation Multiplexer  sim_sel=1  hw_sel=2
  Simulation Multiplexer1 : xbsIndex_r3/Simulation Multiplexer  sim_sel=1  hw_sel=2
  ZBT SRAM 32Bit Generation : Subsystem
  ZBT SRAM 32Bit Simulation : Subsystem
  q : Outport
  qv : Outport  Port=2
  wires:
  r/1 -> ZBT SRAM 32Bit Generation/4(r), ZBT SRAM 32Bit Simulation/4(r)
  w/1 -> ZBT SRAM 32Bit Generation/3(w), ZBT SRAM 32Bit Simulation/3(w)
  a/1 -> ZBT SRAM 32Bit Generation/2(a), ZBT SRAM 32Bit Simulation/2(a)
  d/1 -> ZBT SRAM 32Bit Generation/1(d), ZBT SRAM 32Bit Simulation/1(d)
  ZBT SRAM 32Bit Simulation/2(qv) -> Simulation Multiplexer1/1
  ZBT SRAM 32Bit Simulation/1(q) -> Simulation Multiplexer/1
  ZBT SRAM 32Bit Generation/1(q) -> Simulation Multiplexer/2
  ZBT SRAM 32Bit Generation/2(qv) -> Simulation Multiplexer1/2
  Simulation Multiplexer1/1 -> qv/1
  Simulation Multiplexer/1 -> q/1
  be/1 -> ZBT SRAM 32Bit Simulation/5(be), ZBT SRAM 32Bit Generation/5(be)

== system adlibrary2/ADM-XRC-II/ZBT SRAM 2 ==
  d : Inport  Port=1  LatchInput=off
  a : Inport  Port=2  LatchInput=off
  w : Inport  Port=3  LatchInput=off
  r : Inport  Port=4  LatchInput=off
  be : Inport  Port=5  LatchInput=off
  Simulation Multiplexer : xbsIndex_r3/Simulation Multiplexer  sim_sel=1  hw_sel=2
  Simulation Multiplexer1 : xbsIndex_r3/Simulation Multiplexer  sim_sel=1  hw_sel=2
  ZBT SRAM 32Bit Generation : Subsystem
  ZBT SRAM 32Bit Simulation : Subsystem
  q : Outport
  qv : Outport  Port=2
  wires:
  r/1 -> ZBT SRAM 32Bit Generation/4(r), ZBT SRAM 32Bit Simulation/4(r)
  w/1 -> ZBT SRAM 32Bit Generation/3(w), ZBT SRAM 32Bit Simulation/3(w)
  a/1 -> ZBT SRAM 32Bit Generation/2(a), ZBT SRAM 32Bit Simulation/2(a)
  d/1 -> ZBT SRAM 32Bit Generation/1(d), ZBT SRAM 32Bit Simulation/1(d)
  ZBT SRAM 32Bit Simulation/2(qv) -> Simulation Multiplexer1/1
  ZBT SRAM 32Bit Simulation/1(q) -> Simulation Multiplexer/1
  ZBT SRAM 32Bit Generation/1(q) -> Simulation Multiplexer/2
  ZBT SRAM 32Bit Generation/2(qv) -> Simulation Multiplexer1/2
  Simulation Multiplexer1/1 -> qv/1
  Simulation Multiplexer/1 -> q/1
  be/1 -> ZBT SRAM 32Bit Simulation/5(be), ZBT SRAM 32Bit Generation/5(be)

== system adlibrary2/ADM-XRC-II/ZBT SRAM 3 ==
  d : Inport  Port=1  LatchInput=off
  a : Inport  Port=2  LatchInput=off
  w : Inport  Port=3  LatchInput=off
  r : Inport  Port=4  LatchInput=off
  be : Inport  Port=5  LatchInput=off
  Simulation Multiplexer : xbsIndex_r3/Simulation Multiplexer  sim_sel=1  hw_sel=2
  Simulation Multiplexer1 : xbsIndex_r3/Simulation Multiplexer  sim_sel=1  hw_sel=2
  ZBT SRAM 32Bit Generation : Subsystem
  ZBT SRAM 32Bit Simulation : Subsystem
  q : Outport
  qv : Outport  Port=2
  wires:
  r/1 -> ZBT SRAM 32Bit Generation/4(r), ZBT SRAM 32Bit Simulation/4(r)
  w/1 -> ZBT SRAM 32Bit Generation/3(w), ZBT SRAM 32Bit Simulation/3(w)
  a/1 -> ZBT SRAM 32Bit Generation/2(a), ZBT SRAM 32Bit Simulation/2(a)
  d/1 -> ZBT SRAM 32Bit Generation/1(d), ZBT SRAM 32Bit Simulation/1(d)
  ZBT SRAM 32Bit Simulation/2(qv) -> Simulation Multiplexer1/1
  ZBT SRAM 32Bit Simulation/1(q) -> Simulation Multiplexer/1
  ZBT SRAM 32Bit Generation/1(q) -> Simulation Multiplexer/2
  ZBT SRAM 32Bit Generation/2(qv) -> Simulation Multiplexer1/2
  Simulation Multiplexer1/1 -> qv/1
  Simulation Multiplexer/1 -> q/1
  be/1 -> ZBT SRAM 32Bit Simulation/5(be), ZBT SRAM 32Bit Generation/5(be)

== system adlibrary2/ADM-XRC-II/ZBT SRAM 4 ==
  d : Inport  Port=1  LatchInput=off
  a : Inport  Port=2  LatchInput=off
  w : Inport  Port=3  LatchInput=off
  r : Inport  Port=4  LatchInput=off
  be : Inport  Port=5  LatchInput=off
  Simulation Multiplexer : xbsIndex_r3/Simulation Multiplexer  sim_sel=1  hw_sel=2
  Simulation Multiplexer1 : xbsIndex_r3/Simulation Multiplexer  sim_sel=1  hw_sel=2
  ZBT SRAM 32Bit Generation : Subsystem
  ZBT SRAM 32Bit Simulation : Subsystem
  q : Outport
  qv : Outport  Port=2
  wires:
  r/1 -> ZBT SRAM 32Bit Generation/4(r), ZBT SRAM 32Bit Simulation/4(r)
  w/1 -> ZBT SRAM 32Bit Generation/3(w), ZBT SRAM 32Bit Simulation/3(w)
  a/1 -> ZBT SRAM 32Bit Generation/2(a), ZBT SRAM 32Bit Simulation/2(a)
  d/1 -> ZBT SRAM 32Bit Generation/1(d), ZBT SRAM 32Bit Simulation/1(d)
  ZBT SRAM 32Bit Simulation/2(qv) -> Simulation Multiplexer1/1
  ZBT SRAM 32Bit Simulation/1(q) -> Simulation Multiplexer/1
  ZBT SRAM 32Bit Generation/1(q) -> Simulation Multiplexer/2
  ZBT SRAM 32Bit Generation/2(qv) -> Simulation Multiplexer1/2
  Simulation Multiplexer1/1 -> qv/1
  Simulation Multiplexer/1 -> q/1
  be/1 -> ZBT SRAM 32Bit Simulation/5(be), ZBT SRAM 32Bit Generation/5(be)

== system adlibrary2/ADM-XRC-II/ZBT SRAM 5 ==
  d : Inport  Port=1  LatchInput=off
  a : Inport  Port=2  LatchInput=off
  w : Inport  Port=3  LatchInput=off
  r : Inport  Port=4  LatchInput=off
  be : Inport  Port=5  LatchInput=off
  Simulation Multiplexer : xbsIndex_r3/Simulation Multiplexer  sim_sel=1  hw_sel=2
  Simulation Multiplexer1 : xbsIndex_r3/Simulation Multiplexer  sim_sel=1  hw_sel=2
  ZBT SRAM 32Bit Generation : Subsystem
  ZBT SRAM 32Bit Simulation : Subsystem
  q : Outport
  qv : Outport  Port=2
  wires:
  r/1 -> ZBT SRAM 32Bit Generation/4(r), ZBT SRAM 32Bit Simulation/4(r)
  w/1 -> ZBT SRAM 32Bit Generation/3(w), ZBT SRAM 32Bit Simulation/3(w)
  a/1 -> ZBT SRAM 32Bit Generation/2(a), ZBT SRAM 32Bit Simulation/2(a)
  d/1 -> ZBT SRAM 32Bit Generation/1(d), ZBT SRAM 32Bit Simulation/1(d)
  ZBT SRAM 32Bit Simulation/2(qv) -> Simulation Multiplexer1/1
  ZBT SRAM 32Bit Simulation/1(q) -> Simulation Multiplexer/1
  ZBT SRAM 32Bit Generation/1(q) -> Simulation Multiplexer/2
  ZBT SRAM 32Bit Generation/2(qv) -> Simulation Multiplexer1/2
  Simulation Multiplexer1/1 -> qv/1
  Simulation Multiplexer/1 -> q/1
  be/1 -> ZBT SRAM 32Bit Simulation/5(be), ZBT SRAM 32Bit Generation/5(be)

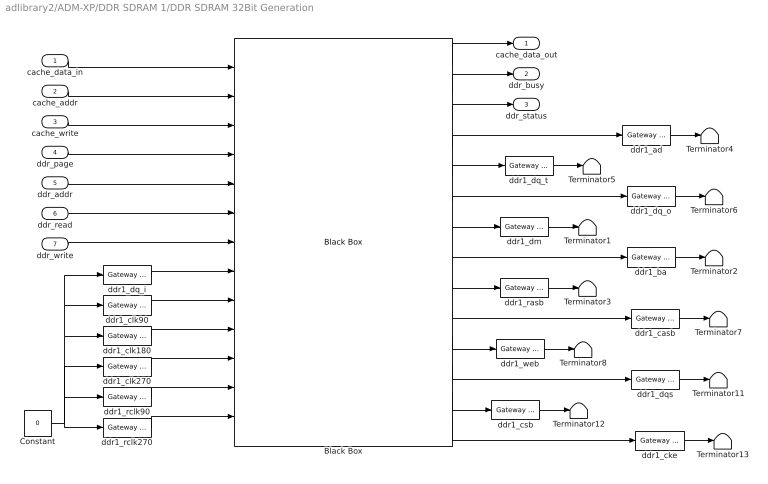
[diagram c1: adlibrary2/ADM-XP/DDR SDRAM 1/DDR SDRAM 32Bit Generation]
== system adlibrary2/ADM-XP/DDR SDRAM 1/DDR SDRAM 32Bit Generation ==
  cache_data_in : Inport  Port=1  LatchInput=off
  cache_addr : Inport  Port=2  LatchInput=off
  cache_write : Inport  Port=3  LatchInput=off
  ddr_page : Inport  Port=4  LatchInput=off
  ddr_addr : Inport  Port=5  LatchInput=off
  ddr_read : Inport  Port=6  LatchInput=off
  ddr_write : Inport  Port=7  LatchInput=off
  Black Box : xbsIndex_r3/Black Box  init_code=ddr32_config  sim_method=Inactive  show_param=on
  Constant : Constant  Value=0
  Terminator{1..8,11..13} (11 alike) : Terminator
  ddr1_ad : xbsIndex_r3/Gateway Out  hdl_port=on  timing_constraint=None  locs_specified=off  LOCs={}  needs_fixed_name=off  show_param=off
  ddr1_ba : xbsIndex_r3/Gateway Out  hdl_port=on  timing_constraint=None  locs_specified=off  LOCs={}  needs_fixed_name=off  show_param=off
  ddr1_casb : xbsIndex_r3/Gateway Out  hdl_port=on  timing_constraint=None  locs_specified=off  LOCs={}  needs_fixed_name=off  show_param=off
  ddr1_cke : xbsIndex_r3/Gateway Out  hdl_port=on  timing_constraint=None  locs_specified=off  LOCs={}  needs_fixed_name=off  show_param=off
  ddr1_clk180 : xbsIndex_r3/Gateway In  arith_type=Boolean  n_bits=64  bin_pt=0  quantization=Truncate  overflow=Wrap  period=1  timing_constraint=None  locs_specified=off  LOCs={}  needs_fixed_name=off  dbl_ovrd=off  show_param=off
  ddr1_clk270 : xbsIndex_r3/Gateway In  arith_type=Boolean  n_bits=64  bin_pt=0  quantization=Truncate  overflow=Wrap  period=1  timing_constraint=None  locs_specified=off  LOCs={}  needs_fixed_name=off  dbl_ovrd=off  show_param=off
  ddr1_clk90 : xbsIndex_r3/Gateway In  arith_type=Boolean  n_bits=64  bin_pt=0  quantization=Truncate  overflow=Wrap  period=1  timing_constraint=None  locs_specified=off  LOCs={}  needs_fixed_name=off  dbl_ovrd=off  show_param=off
  ddr1_csb : xbsIndex_r3/Gateway Out  hdl_port=on  timing_constraint=None  locs_specified=off  LOCs={}  needs_fixed_name=off  show_param=off
  ddr1_dm : xbsIndex_r3/Gateway Out  hdl_port=on  timing_constraint=None  locs_specified=off  LOCs={}  needs_fixed_name=off  show_param=off
  ddr1_dq_i : xbsIndex_r3/Gateway In  arith_type=Unsigned  n_bits=32  bin_pt=0  quantization=Truncate  overflow=Wrap  period=1  timing_constraint=None  locs_specified=off  LOCs={}  needs_fixed_name=off  dbl_ovrd=off  show_param=off
  ddr1_dq_o : xbsIndex_r3/Gateway Out  hdl_port=on  timing_constraint=None  locs_specified=off  LOCs={}  needs_fixed_name=off  show_param=off
  ddr1_dq_t : xbsIndex_r3/Gateway Out  hdl_port=on  timing_constraint=None  locs_specified=off  LOCs={}  needs_fixed_name=off  show_param=off
  ddr1_dqs : xbsIndex_r3/Gateway Out  hdl_port=on  timing_constraint=None  locs_specified=off  LOCs={}  needs_fixed_name=off  show_param=off
  ddr1_rasb : xbsIndex_r3/Gateway Out  hdl_port=on  timing_constraint=None  locs_specified=off  LOCs={}  needs_fixed_name=off  show_param=off
  ddr1_rclk270 : xbsIndex_r3/Gateway In  arith_type=Boolean  n_bits=64  bin_pt=0  quantization=Truncate  overflow=Wrap  period=1  timing_constraint=None  locs_specified=off  LOCs={}  needs_fixed_name=off  dbl_ovrd=off  show_param=off
  ddr1_rclk90 : xbsIndex_r3/Gateway In  arith_type=Boolean  n_bits=64  bin_pt=0  quantization=Truncate  overflow=Wrap  period=1  timing_constraint=None  locs_specified=off  LOCs={}  needs_fixed_name=off  dbl_ovrd=off  show_param=off
  ddr1_web : xbsIndex_r3/Gateway Out  hdl_port=on  timing_constraint=None  locs_specified=off  LOCs={}  needs_fixed_name=off  show_param=off
  cache_data_out : Outport
  ddr_busy : Outport  Port=2
  ddr_status : Outport  Port=3
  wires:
  Black Box/14 -> ddr1_cke/1
  ddr1_cke/1 -> Terminator13/1
  Black Box/13 -> ddr1_csb/1
  ddr1_csb/1 -> Terminator12/1
  ddr1_dqs/1 -> Terminator11/1
  Black Box/11 -> ddr1_web/1
  ddr1_web/1 -> Terminator8/1
  Black Box/10 -> ddr1_casb/1
  ddr1_casb/1 -> Terminator7/1
  Black Box/9 -> ddr1_rasb/1
  ddr1_rasb/1 -> Terminator3/1
  Black Box/8 -> ddr1_ba/1
  ddr1_ba/1 -> Terminator2/1
  Black Box/7 -> ddr1_dm/1
  ddr1_dm/1 -> Terminator1/1
  Black Box/6 -> ddr1_dq_o/1
  ddr1_dq_o/1 -> Terminator6/1
  Black Box/5 -> ddr1_dq_t/1
  ddr1_dq_t/1 -> Terminator5/1
  ddr1_ad/1 -> Terminator4/1
  Black Box/4 -> ddr1_ad/1
  Black Box/3 -> ddr_status/1
  Black Box/2 -> ddr_busy/1
  Black Box/1 -> cache_data_out/1
  ddr_write/1 -> Black Box/7
  ddr_read/1 -> Black Box/6
  ddr_addr/1 -> Black Box/5
  ddr_page/1 -> Black Box/4
  cache_write/1 -> Black Box/3
  cache_addr/1 -> Black Box/2
  cache_data_in/1 -> Black Box/1
  ddr1_dq_i/1 -> Black Box/8
  Constant/1 -> ddr1_dq_i/1, ddr1_clk90/1, ddr1_clk180/1, ddr1_rclk270/1, ddr1_clk270/1, ddr1_rclk90/1
  Black Box/12 -> ddr1_dqs/1
  ddr1_clk90/1 -> Black Box/9
  ddr1_clk180/1 -> Black Box/10
  ddr1_clk270/1 -> Black Box/11
  ddr1_rclk90/1 -> Black Box/12
  ddr1_rclk270/1 -> Black Box/13

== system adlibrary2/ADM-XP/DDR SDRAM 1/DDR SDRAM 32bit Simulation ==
  cache_data_in : Inport  Port=1  LatchInput=off
  cache_addr : Inport  Port=2  LatchInput=off
  cache_write : Inport  Port=3  LatchInput=off
  ddr_page : Inport  Port=4  LatchInput=off
  ddr_addr : Inport  Port=5  LatchInput=off
  ddr_read : Inport  Port=6  LatchInput=off
  ddr_write : Inport  Port=7  LatchInput=off
  Disregard Subsystem : xbsIndex_r3/Disregard Subsystem  Tag=discardX
  S-Function : S-Function  FunctionName=ddr32  Parameters=memsize
  Subsystem : adlibrary2/ADM-XRC-II/XRM DDR SDRAM /DDR SDRAM 64bit Simulation/Subsystem
  gi{0..6} (7 alike) : xbsIndex_r3/Gateway Out  hdl_port=off  timing_constraint=None  locs_specified=off  LOCs={}  needs_fixed_name=off  show_param=off
  cache_data_out : Outport
  ddr_busy : Outport  Port=2
  ddr_status : Outport  Port=3
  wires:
  cache_data_in/1 -> gi0/1
  cache_addr/1 -> gi1/1
  cache_write/1 -> gi2/1
  ddr_page/1 -> gi3/1
  ddr_addr/1 -> gi4/1
  ddr_read/1 -> gi5/1
  ddr_write/1 -> gi6/1
  gi0/1 -> S-Function/1
  gi1/1 -> S-Function/2
  gi2/1 -> S-Function/3
  gi3/1 -> S-Function/4
  gi4/1 -> S-Function/5
  gi5/1 -> S-Function/6
  gi6/1 -> S-Function/7
  S-Function/3 -> Subsystem/3
  S-Function/2 -> Subsystem/2
  S-Function/1 -> Subsystem/1
  Subsystem/1 -> cache_data_out/1
  Subsystem/2 -> ddr_busy/1
  Subsystem/3 -> ddr_status/1
